| TI DM646x IBIS MODEL with DDR2
[IBIS Ver]   3.2
[File Name]   sprm277e.ibs
[File Rev]   0.2
[Date]   April 30, 2009
[Source]   TI
[Disclaimer]   Please be aware that in the absence of a written agreement
|   Texas Instruments(TI) assumes no liability for:
|   (1) The accuracy of the IBIS models provided to your company
|   (2) The proper functioning of these Models in your design
|   or for any resulting applications
|   (3) Infringement of patents, copyrights or intellectual
|   property rights resulting from your use of these
|   models.
|   TI provides IBIS Models as a service to our customers and
|   therefore reserves the right to limit distribution of the
|   Models.
[Copyright]   Property of Texas Instruments Incorporated.
|   Unauthorized reproduction and/or distribution is strictly.
|   prohibited.
|   This product is protected under copyright law and trade
|   secret law as an unpublished work.
|   Created 2007,(C) Copyright 1999-2007,
|   Texas Instruments Incorporated., All Rights Reserved.
|   These commodities are under the U.S. Government
|   distribution license control. As such,they are not to be
|   re-exported without the prior approval of the U.S.
|   Department of Commerce.
[Notes]
| Component   DM646x
[Component]   DM646x
[Manufacturer]   Texas Instruments
[Package]
| variable   typ   min   max
R_pkg   2.45454E-01   5.83181E-02   4.83686E-01
L_pkg   2.60207E-09   1.54140E-09   4.10250E-09
C_pkg   1.55780E-12   1.08555E-12   2.17328E-12
[Pin] signal_name   model_name   R_pin   L_pin   C_pin
A11   PCI_INTBN   BPCI33TPUFZP18   2.7877E-01 2.7673E-09 1.6313E-12
C11   PCI_INTAN   BPCI33TPUFZP18   1.8694E-01 2.2210E-09 1.3859E-12
D11   PCI_INTCN   BPCI33TPUFZP18   1.3871E-01 1.9025E-09 1.2538E-12
B11   GP05_INT05   BPCI33TPDFZP18   2.3300E-01 2.5519E-09 1.4959E-12
A12   GP07_INT07   BPCI33TPDFZP18   2.7619E-01 2.8667E-09 1.6467E-12
A10   PCI_CLK   BPCI33TPUFZP18   2.6854E-01 2.8128E-09 1.5917E-12
C10   PCI_RSTN   BPCI33TPDFZP18   1.5935E-01 2.1439E-09 1.3432E-12
B12   TCLK   IQ33STCKP18PUSR50   2.4188E-01 2.5826E-09 1.5351E-12
B10   PCI_REQ2N   BPCI33TPDFZP18   2.2910E-01 2.4910E-09 1.4928E-12
E11   GP06_INT06   BPCI33TPDFZP18   8.4748E-02 1.6414E-09 1.1002E-12
D12   TMS   IT33SHYPUFZP18   1.4649E-01 1.9445E-09 1.2763E-12
D10   PCI_GNTN   BPCI33TPUFZP18   1.5951E-01 2.0675E-09 1.3045E-12
E10   PCI_GNT2N   BPCI33TPUFZP18   9.3986E-02 1.6149E-09 1.1264E-12
E12   TRSTN   IT33SHYPDFZP18   1.1940E-01 1.7969E-09 1.2210E-12
C12   RTCK   OT3350CSFZP18   2.0113E-01 2.2992E-09 1.4287E-12
|C15  VSS_DEV   GND   5.5062E-02 1.6374E-09 1.9419E-12
B15   X1DEV_CKINDEV   NC   2.3651E-01 2.4675E-09 1.5117E-12
A15   X2DEV   NC   2.9679E-01 2.8758E-09 1.6904E-12
|D15  VDDS   POWER   7.5928E-02 1.7083E-09 1.8787E-12
|A16  VSSA2   GND   7.2873E-02 1.8878E-09 2.4529E-12
|C14  VSSA   GND   6.6017E-02 1.7036E-09 2.0833E-12
|C16  VSSS2   GND   6.3900E-02 1.5792E-09 1.9390E-12
|B14  VDDA18V   POWER   6.7389E-02 1.6921E-09 2.1872E-12
|D16  VDDS2   POWER   7.2580E-02 1.6472E-09 1.7765E-12
|B16  VDDA18V2   POWER   7.9345E-02 1.7827E-09 2.2027E-12
|C17  VSS_AUX   GND   8.3082E-02 1.7375E-09 1.9680E-12
B17   X1AUX_CKINAUX   NC   2.5695E-01 2.6223E-09 1.5724E-12
A17   X2AUX   NC   2.8397E-01 2.8078E-09 1.6441E-12
|E16  VDD5   POWER   9.4062E-02 1.6917E-09 1.5592E-12
D17   PORN   IT33SHYPUFZP18   1.7201E-01 2.1219E-09 1.3281E-12
C18   USB_VSSREF   NC   5.8318E-02 1.6295E-09 1.9812E-12
B18   USB_DRVVBUS   OPERATIONAL_MODE   2.5336E-01 2.7069E-09 1.6138E-12
|P23  VREF_DDR   POWER   4.9018E-02 1.3868E-09 7.8262E-12
N23   DDR_A14   BSHTLDVGPBFZIDID   2.8514E-01 2.8886E-09 1.6855E-12
N22   DDR_A09   BSHTLDVGPBFZIDID   2.2962E-01 2.4944E-09 1.5400E-12
N21   DDR_A05   BSHTLDVGPBFZIDID   1.9430E-01 2.3197E-09 1.4271E-12
R23   DDR_A01   BSHTLDVGPBFZIDID   3.7618E-01 3.6698E-09 1.8926E-12
Y21   DDR_D29   BSHTLDVGPBFZIDID   3.0072E-01 2.8974E-09 1.6783E-12
H22   DDR_D15   BSHTLDVGPBFZIDID   4.3087E-01 3.6600E-09 2.0046E-12
U20   DDR_DQS3   BSHTLDVGPBFZIDID   2.8732E-01 2.8089E-09 1.5764E-12
G22   DDR_D13   BSHTLDVGPBFZIDID   4.4213E-01 3.7401E-09 1.9738E-12
T23   DDR_A10   BSHTLDVGPBFZIDID   3.4959E-01 3.4591E-09 1.8147E-12
A2   THERMAL_P   NC   3.3115E-01 3.1439E-09 1.9476E-12
A1   THERMAL_N   NC   3.7687E-01 3.5180E-09 1.9528E-12
B3   PCI_DEVSELN   BPCI33TPUFZP18   3.0811E-01 2.9904E-09 1.7689E-12
A3   PCI_IRDYN   BPCI33TPUFZP18   3.6344E-01 3.2863E-09 1.8773E-12
C3   PCI_PERRN   BPCI33TPUFZP18   2.6286E-01 2.6646E-09 1.6213E-12
B2   PCI_SERRN   BPCI33TPUFZP18   2.8503E-01 2.8397E-09 1.7099E-12
D5   PCI_STOPN   BPCI33TPUFZP18   1.7666E-01 2.1759E-09 1.3763E-12
C1   PCI_AD14   BPCI33TPDFZP18   3.3204E-01 3.1677E-09 1.7799E-12
C4   PCI_CBE2N   BPCI33TPUFZP18   2.8951E-01 2.9542E-09 1.6700E-12
B4   PCI_AD17   BPCI33TPDFZP18   3.0308E-01 2.9750E-09 1.7299E-12
D4   PCI_PAR   BPCI33TPUFZP18   1.9363E-01 2.2404E-09 1.4282E-12
C2   PCI_CBE1N   BPCI33TPUFZP18   2.6565E-01 2.7844E-09 1.6478E-12
D2   PCI_AD10   BPCI33TPDFZP18   2.7296E-01 2.8166E-09 1.6458E-12
E5   PCI_AD15   BPCI33TPDFZP18   1.3925E-01 1.9027E-09 1.2655E-12
D3   PCI_AD12   BPCI33TPDFZP18   2.4623E-01 2.6009E-09 1.5479E-12
D6   PCI_FRAMEN   BPCI33TPUFZP18   1.8217E-01 2.2248E-09 1.3886E-12
C5   PCI_AD21   BPCI33TPDFZP18   2.8181E-01 2.8221E-09 1.6211E-12
C6   PCI_AD16   BPCI33TPDFZP18   2.1425E-01 2.4965E-09 1.4441E-12
E4   PCI_AD13   BPCI33TPDFZP18   1.6213E-01 2.0692E-09 1.3389E-12
E6   PCI_TRDYN   BPCI33TPUFZP18   1.0725E-01 1.7677E-09 1.1929E-12
A4   PCI_AD19   BPCI33TPDFZP18   3.8327E-01 3.4263E-09 1.9108E-12
E7   PCI_AD18   BPCI33TPDFZP18   1.2702E-01 1.7420E-09 1.2068E-12
D7   PCI_AD20   BPCI33TPDFZP18   1.5322E-01 2.0190E-09 1.2765E-12
F5   PCI_AD9   BPCI33TPDFZP18   1.4050E-01 1.9648E-09 1.2543E-12
C7   PCI_AD22   BPCI33TPDFZP18   1.8238E-01 2.1596E-09 1.4090E-12
B5   PCI_AD23   BPCI33TPDFZP18   2.9356E-01 2.8622E-09 1.7076E-12
B6   PCI_AD25   BPCI33TPDFZP18   2.9546E-01 2.8485E-09 1.7200E-12
A5   PCI_CBE3N   BPCI33TPUFZP18   3.6680E-01 3.3978E-09 1.9010E-12
E8   PCI_IDSEL   BPCI33TPUFZP18   1.2603E-01 1.8511E-09 1.2174E-12
D8   PCI_AD24   BPCI33TPDFZP18   1.4545E-01 1.9034E-09 1.2897E-12
C8   PCI_AD26   BPCI33TPDFZP18   1.9932E-01 2.2035E-09 1.4169E-12
B8   PCI_AD29   BPCI33TPDFZP18   2.2504E-01 2.4923E-09 1.5032E-12
A6   PCI_AD27   BPCI33TPDFZP18   3.4528E-01 3.2406E-09 1.8202E-12
E9   PCI_GNT1N   BPCI33TPDFZP18   1.0641E-01 1.7227E-09 1.1832E-12
D9   PCI_AD28   BPCI33TPDFZP18   1.7577E-01 2.1341E-09 1.3584E-12
C9   PCI_AD30   BPCI33TPDFZP18   1.9116E-01 2.2644E-09 1.3919E-12
A8   PCI_AD31   BPCI33TPDFZP18   2.9816E-01 2.8914E-09 1.6888E-12
B9   PCI_REQN   BPCI33TPUFZP18   2.2823E-01 2.4067E-09 1.5054E-12
A9   PCI_REQ1N   BPCI33TPDFZP18   2.4922E-01 2.7180E-09 1.5936E-12
A13   EMU0   BT3350CSHYPUFZP18   2.8486E-01 2.8884E-09 1.6409E-12
B13   EMU1   BT3350CSHYPUFZP18   2.5408E-01 2.7080E-09 1.5863E-12
C13   CLKOUT0   OT3350BSFZP18   2.1075E-01 2.5326E-09 1.4228E-12
D13   TDO   OT3350CSFZP18   1.9701E-01 2.3477E-09 1.4279E-12
E13   TDI   IT33SHYPUFZP18   1.2685E-01 1.9618E-09 1.2659E-12
D14   AMUX   NC   6.0907E-02 1.5939E-09 1.7516E-12
|E14  VSSS1   GND   5.5579E-02 1.5715E-09 1.4300E-12
|E15  VDD6   POWER   6.3533E-02 1.5903E-09 1.5396E-12
A19   USB_DP   DPDM   2.9913E-01 2.8266E-09 1.7243E-12
|E17  VDDA_12LDO   POWER   4.8724E-02 1.4146E-09 1.4594E-12
|G16  VPP   POWER   1.4716E-02 9.8859E-10 2.0313E-12
D18   USB_R1   NC   1.7146E-01 2.1995E-09 1.3651E-12
C20   DDR_D02   BSHTLDVGPBFZIDID   3.7216E-01 3.2805E-09 1.7796E-12
A20   USB_DN   DPDM   2.9706E-01 2.8346E-09 1.7381E-12
D20   DDR_D01   BSHTLDVGPBFZIDID   3.3792E-01 3.1510E-09 1.7608E-12
|E18  VDD_18UPHY   POWER   5.6087E-02 1.5095E-09 1.5146E-12
|F18  VDDA_33UPHY   POWER   3.8147E-02 1.3788E-09 1.3634E-12
F20   DDR_DQM0   BSHTLDVGPBFZIDID   3.4058E-01 3.0257E-09 1.7935E-12
A22   IFORCE   NC   3.8507E-01 3.4309E-09 1.9972E-12
B21   DDR_D03   BSHTLDVGPBFZIDID   3.8767E-01 3.4318E-09 1.9469E-12
G20   DDR_D04   BSHTLDVGPBFZIDID   3.4303E-01 3.0700E-09 1.7241E-12
E20   DDR_DQSN0   BSHTLDVGPBFZIDID   3.5451E-01 3.1555E-09 1.7460E-12
A23   VSENSE   NC   4.3154E-01 3.8929E-09 2.0758E-12
C21   DDR_D00   BSHTLDVGPBFZIDID   3.8272E-01 3.2914E-09 1.8910E-12
B22   DDR_D09   BSHTLDVGPBFZIDID   4.8369E-01 4.1025E-09 2.1733E-12
C23   DDR_D08   BSHTLDVGPBFZIDID   4.3765E-01 3.7508E-09 2.0793E-12
C22   DDR_D10   BSHTLDVGPBFZIDID   4.3926E-01 3.6854E-09 2.0784E-12
J19   DDR_DQGATE0   BSHTLDVGPBFZIDID   1.3943E-01 1.8775E-09 1.2336E-12
D21   DDR_DQS0   BSHTLDVGPBFZIDID   3.5612E-01 3.2791E-09 1.8411E-12
F21   DDR_D05   BSHTLDVGPBFZIDID   3.5077E-01 3.1080E-09 1.8262E-12
G21   DDR_D06   BSHTLDVGPBFZIDID   3.4698E-01 3.1246E-09 1.7646E-12
D22   DDR_DQS1   BSHTLDVGPBFZIDID   4.4339E-01 3.7215E-09 2.1383E-12
H20   DDR_D07   BSHTLDVGPBFZIDID   3.4601E-01 3.0269E-09 1.7012E-12
J21   DDR_DQGATE1   BSHTLDVGPBFZIDID   1.6504E-01 2.1300E-09 1.3912E-12
H21   DDR_A13   BSHTLDVGPBFZIDID   2.6986E-01 2.7281E-09 1.6286E-12
F22   DDR_DQM1   BSHTLDVGPBFZIDID   4.2218E-01 3.5920E-09 2.0151E-12
J20   DDR_CSN   BSHTLDVGPBFZIDID   2.0809E-01 2.4992E-09 1.5659E-12
K20   DDR_ODT0   BSHTLDVGPBFZIDID   1.3671E-01 1.9192E-09 1.2745E-12
K19   DDR_RASN   BSHTLDVGPBFZIDID   1.3844E-01 2.0285E-09 1.3514E-12
J22   DDR_A04   BSHTLDVGPBFZIDID   2.5719E-01 2.6382E-09 1.6209E-12
D23   DDR_DQSN1   BSHTLDVGPBFZIDID   4.4173E-01 3.6954E-09 2.1371E-12
E23   DDR_D11   BSHTLDVGPBFZIDID   4.3505E-01 3.7028E-09 1.9933E-12
F23   DDR_D12   BSHTLDVGPBFZIDID   4.4355E-01 3.6991E-09 2.0659E-12
G23   DDR_D14   BSHTLDVGPBFZIDID   4.2279E-01 3.7370E-09 2.0122E-12
H23   DDR_A00   BSHTLDVGPBFZIDID   3.1449E-01 3.0248E-09 1.7505E-12
J23   DDR_A08   BSHTLDVGPBFZIDID   3.4902E-01 3.3817E-09 1.8271E-12
L20   DDR_WEN   BSHTLDVGPBFZIDID   1.7445E-01 2.1296E-09 1.3326E-12
L21   DDR_CASN   BSHTLDVGPBFZIDID   1.9727E-01 2.2693E-09 1.4121E-12
L19   DDR_REFP   NC   1.3252E-01 2.1619E-09 1.2826E-12
K23   DDR_A11   BSHTLDVGPBFZIDID   2.7410E-01 2.7849E-09 1.6432E-12
M22   DDR_A06   BSHTLDVGPBFZIDID   2.3631E-01 2.6236E-09 1.5578E-12
L22   DDR_A02   BSHTLDVGPBFZIDID   2.4786E-01 2.9281E-09 1.5341E-12
M21   DDR_BA1   BSHTLDVGPBFZIDID   1.7634E-01 2.2453E-09 1.3659E-12
M20   DDR_CKE   BSHTLDVGPBFZIDID   1.6773E-01 2.1873E-09 1.3066E-12
L23   DDR_CLKN   BSHTLDVGPBFZIDID   2.9719E-01 3.0043E-09 1.6909E-12
M23   DDR_CLK   BSHTLDVGPBFZIDID   2.9064E-01 2.8534E-09 1.7072E-12
M19   DDR_REFN   NC   9.8133E-02 1.6910E-09 1.1266E-12
R22   DDR_A03   BSHTLDVGPBFZIDID   2.7119E-01 2.8434E-09 1.6357E-12
T22   DDR_D17   BSHTLDVGPBFZIDID   3.9328E-01 3.4903E-09 1.9637E-12
N19   DDR_BA0   BSHTLDVGPBFZIDID   7.9436E-02 1.5414E-09 1.0856E-12
N20   DDR_A07   BSHTLDVGPBFZIDID   1.3620E-01 2.0966E-09 1.2215E-12
P20   DDR_A12   BSHTLDVGPBFZIDID   1.4662E-01 1.9794E-09 1.2429E-12
R21   DDR_DQGATE3   BSHTLDVGPBFZIDID   1.9255E-01 2.2141E-09 1.3949E-12
U23   DDR_D18   BSHTLDVGPBFZIDID   4.0960E-01 3.6369E-09 1.9140E-12
U22   DDR_D16   BSHTLDVGPBFZIDID   4.2102E-01 3.8021E-09 1.9612E-12
P19   DDR_BA2   BSHTLDVGPBFZIDID   1.4495E-01 2.0123E-09 1.2598E-12
R19   DDR_DQGATE2   BSHTLDVGPBFZIDID   1.4044E-01 1.8898E-09 1.1869E-12
R20   DDR_D25   BSHTLDVGPBFZIDID   2.8920E-01 2.7835E-09 1.6410E-12
Y23   DDR_DQM2   BSHTLDVGPBFZIDID   4.4716E-01 4.0407E-09 2.1157E-12
T21   DDR_D26   BSHTLDVGPBFZIDID   2.8616E-01 2.7532E-09 1.6110E-12
AA23  DDR_D20   BSHTLDVGPBFZIDID   4.4661E-01 3.9010E-09 2.1348E-12
W23   DDR_DQSN2   BSHTLDVGPBFZIDID   4.1680E-01 3.6580E-09 2.0554E-12
Y22   DDR_D22   BSHTLDVGPBFZIDID   4.1015E-01 3.5365E-09 2.0298E-12
AA22  DDR_D21   BSHTLDVGPBFZIDID   4.5800E-01 4.0009E-09 2.1196E-12
V23   DDR_D19   BSHTLDVGPBFZIDID   4.0434E-01 3.6008E-09 1.9715E-12
V22   DDR_DQS2   BSHTLDVGPBFZIDID   4.1978E-01 3.6565E-09 1.9620E-12
U21   DDR_D27   BSHTLDVGPBFZIDID   2.9025E-01 2.7701E-09 1.6060E-12
V21   DDR_DQSN3   BSHTLDVGPBFZIDID   2.8454E-01 2.6807E-09 1.6218E-12
AB22  DDR_D23   BSHTLDVGPBFZIDID   4.5536E-01 4.0091E-09 2.1416E-12
AA21  DDR_D28   BSHTLDVGPBFZIDID   3.2699E-01 3.0902E-09 1.6728E-12
AC21  UART2_CTSN   BT3350BSHYPUFZP18   3.3320E-01 3.1564E-09 1.7751E-12
T20   DDR_D24   BSHTLDVGPBFZIDID   2.8107E-01 2.8430E-09 1.6321E-12
V20   DDR_DQM3   BSHTLDVGPBFZIDID   2.9327E-01 2.7837E-09 1.6108E-12
W20   DDR_D30   BSHTLDVGPBFZIDID   2.8787E-01 2.8040E-09 1.6332E-12
Y20   DDR_D31   BSHTLDVGPBFZIDID   2.9876E-01 2.8963E-09 1.6159E-12
AB20  UART2_RXD   OPERATIONAL_MODE   2.6882E-01 2.8323E-09 1.6277E-12
Y18   UART1_RXD   OPERATIONAL_MODE   1.5530E-01 1.9932E-09 1.3127E-12
AA19  UART2_TXD   OPERATIONAL_MODE   2.2431E-01 2.4176E-09 1.4946E-12
W18   PWM1   OT3350BSFZP18   8.4804E-02 1.6219E-09 1.1306E-12
W17   PWM0   OT3350BSFZP18   9.0402E-02 1.5786E-09 1.1118E-12
Y17   UART1_CTSN   BT3350BSHYPUFZP18   1.4102E-01 1.9809E-09 1.2447E-12
Y16   VPIF_DIN11   BT3350DSHYPDFZSCP18  1.4363E-01 1.9195E-09 1.3669E-12
AC20  UART2_RTSN   BT3350BSHYPUFZP18   3.4151E-01 3.2147E-09 1.8048E-12
Y15   VPIF_DIN3   BT3350DSHYPDFZSCP18  1.3560E-01 1.8601E-09 1.2381E-12
AC19  PTSI_CLK   BT3350DSHYPDFZSCP18  3.2733E-01 3.0457E-09 1.7567E-12
AB19  UART1_TXD   OPERATIONAL_MODE   2.7053E-01 2.7661E-09 1.6006E-12
AC18  VPIF_DIN15_VSYNC   BT3350DSHYPDFZSCP18  2.7932E-01 2.8561E-09 1.6429E-12
AA18  UART1_RTSN   BT3350BSHYPUFZP18   1.8570E-01 2.2909E-09 1.3928E-12
AB18  VPIF_CLKIN1   BT3350DSHYPDFZSCP18  2.4542E-01 2.6350E-09 1.5337E-12
AA17  VPIF_DIN14_HSYNC   BT3350DSHYPDFZSCP18  1.9262E-01 2.3298E-09 1.3637E-12
AB17  VPIF_DIN13_FIELD   BT3350DSHYPDFZSCP18  2.5132E-01 2.7150E-09 1.5596E-12
AC17  VPIF_DIN12   BT3350DSHYPDFZSCP18  2.6084E-01 2.7842E-09 1.6075E-12
AA16  VPIF_DIN10   BT3350DSHYPDFZSCP18  1.9516E-01 2.4361E-09 1.3961E-12
AC16  VPIF_DIN8   BT3350DSHYPDFZSCP18  2.6928E-01 2.7639E-09 1.6996E-12
AB16  VPIF_DIN9   BT3350DSHYPDFZSCP18  2.1019E-01 2.4044E-09 1.4676E-12
AA15  VPIF_DIN2   BT3350DSHYPDFZSCP18  1.6289E-01 2.1339E-09 1.4187E-12
AB15  VPIF_DIN1   BT3350DSHYPDFZSCP18  2.2152E-01 2.4260E-09 1.4881E-12
AC15  VPIF_DIN0   BT3350DSHYPDFZSCP18  2.7519E-01 2.7685E-09 1.7276E-12
Y14   VPIF_DIN7   BT3350DSHYPDFZSCP18  1.2325E-01 1.8854E-09 1.2171E-12
AA14  VPIF_DIN6   BT3350DSHYPDFZSCP18  1.9104E-01 2.2307E-09 1.3836E-12
AB14  VPIF_DIN5   BT3350DSHYPDFZSCP18  2.2322E-01 2.4590E-09 1.4752E-12
AC14  VPIF_DIN4   BT3350DSHYPDFZSCP18  2.4866E-01 2.6792E-09 1.5862E-12
AC13  VPIF_CLKIN0   BT3350DSHYPDFZSCP18  2.5976E-01 2.5128E-09 1.6572E-12
AB13  UART0_RXD   IT33SHYPDFZP18   2.1891E-01 2.4350E-09 1.5402E-12
AA13  UART0_RTSN   BT3350BSHYPUFZP18   1.7651E-01 2.1599E-09 1.3503E-12
Y13   UART0_TXD   OPERATIONAL_MODE   1.1551E-01 1.7462E-09 1.1995E-12
AC12  UART0_CTSN   BT3350BSHYPUFZP18   2.7766E-01 2.6877E-09 1.6259E-12
AB11  UART0_DSRN   BT3350BSHYPUFZP18   2.4043E-01 2.4347E-09 1.5251E-12
AA11  UART0_DCDN   BT3350BSHYPUFZP18   1.7124E-01 2.0643E-09 1.3628E-12
AC11  STSI_CLK   BT3350DSHYPDFZSCP18  2.5839E-01 2.6519E-09 1.6141E-12
Y12   UART0_DTRN   BT3350BSHYPUFZP18   1.4024E-01 1.8911E-09 1.2584E-12
AC10  VPIF_CLKO3   OT3350CSFZP18   2.7995E-01 2.7900E-09 1.6256E-12
AB10  VPIF_DOUT11   BT3350DSHYPDFZSCP18  2.3455E-01 2.4754E-09 1.5331E-12
Y11   UART0_RIN   OPERATIONAL_MODE   1.4936E-01 1.9491E-09 1.2751E-12
AA10  VPIF_DOUT10   BT3350DSHYPDFZSCP18  2.0346E-01 2.3261E-09 1.5218E-12
Y10   VPIF_CLKIN2   BT3350DSHYPDFZSCP18  1.2823E-01 1.8376E-09 1.3732E-12
AC9   VPIF_CLKIN3   BT3350DSHYPDFZSCP18  2.9240E-01 2.8708E-09 1.6918E-12
AB9   VPIF_DOUT8   BT3350DSHYPDFZSCP18  2.4640E-01 2.6076E-09 1.6771E-12
AC8   VPIF_DOUT9   BT3350DSHYPDFZSCP18  2.9478E-01 2.9570E-09 1.7786E-12
AB8   VPIF_DOUT15   BT3350DSHYPDFZSCP18  2.5729E-01 2.6739E-09 1.6805E-12
AA9   VPIF_CLKO2   OT3350CSFZP18   2.2390E-01 2.4214E-09 1.6053E-12
Y9   VPIF_DOUT13   BT3350DSHYPDFZSCP18  1.4080E-01 1.9714E-09 1.4233E-12
AC7   VPIF_DOUT14   BT3350DSHYPDFZSCP18  3.1034E-01 3.0264E-09 1.8146E-12
AB7   VPIF_DOUT7   BT3350DSHYPDFZSCP18  2.7625E-01 2.8729E-09 1.6145E-12
AA8   VPIF_DOUT12   BT3350DSHYPDFZSCP18  2.0748E-01 2.2980E-09 1.4394E-12
Y8   VPIF_DOUT2_BTMODE2 BT3350DSHYPDFZSCP18  1.5979E-01 2.0654E-09 1.2868E-12
W8   TOUT0   OPERATIONAL_MODE   1.2111E-01 1.8172E-09 1.1672E-12
AC6   VPIF_DOUT5_PCIEN   BT3350DSHYPDFZSCP18  3.2373E-01 3.1423E-09 1.7568E-12
AB6   VPIF_DOUT3_BTMODE3 BT3350DSHYPDFZSCP18  2.6945E-01 2.7674E-09 1.6270E-12
AA7   VPIF_DOUT4_CS2BW   BT3350DSHYPDFZSCP18  2.3870E-01 2.5626E-09 1.5246E-12
Y7   TIN0   OPERATIONAL_MODE   1.7576E-01 2.1685E-09 1.3360E-12
AC5   VPIF_DOUT6_DSPBOOT BT3350DSHYPDFZSCP18  3.3354E-01 3.1744E-09 1.8243E-12
AA6   TIN1   OPERATIONAL_MODE   2.1716E-01 2.4245E-09 1.4749E-12
AC4   VPIF_DOUT1_BTMODE1 BT3350DSHYPDFZSCP18  3.5677E-01 3.3407E-09 1.8479E-12
AB5   VPIF_DOUT0_BTMODE0 BT3350DSHYPDFZSCP18  2.8554E-01 2.8645E-09 1.6703E-12
AB4   TOUT3   OPERATIONAL_MODE   2.9729E-01 3.0600E-09 1.6692E-12
Y6   TIN2   OPERATIONAL_MODE   1.7426E-01 2.2147E-09 1.3603E-12
W7   TOUT1   OPERATIONAL_MODE   1.5461E-01 2.0530E-09 1.2905E-12
AA5   TOUT2   OPERATIONAL_MODE   2.4354E-01 2.6342E-09 1.5345E-12
AA4   GP02_INT02   OPERATIONAL_MODE   2.5812E-01 2.7070E-09 1.5900E-12
AC3   GP04_INT04   OPERATIONAL_MODE   3.7246E-01 3.4943E-09 1.8744E-12
AB3   GP03_INT03   OPERATIONAL_MODE   3.1393E-01 2.9942E-09 1.7522E-12
W6   RESETN   IT33SHYPUFZP18   1.7245E-01 2.1287E-09 1.2881E-12
Y5   TOUT4   OPERATIONAL_MODE   1.9436E-01 2.3107E-09 1.4284E-12
Y4   MCA0_AFSX   OPERATIONAL_MODE   2.1135E-01 2.3148E-09 1.4788E-12
W5   GP00_INT00   OPERATIONAL_MODE   1.5172E-01 1.9685E-09 1.3059E-12
W4   MCA0_AXR2   OPERATIONAL_MODE   1.8296E-01 2.1469E-09 1.3810E-12
V5   GP01_INT01   OPERATIONAL_MODE   1.6559E-01 2.2628E-09 1.3157E-12
AB2   MCA0_AHCLKR   OPERATIONAL_MODE   3.7868E-01 3.4051E-09 1.9200E-12
AA2   MCA0_ACLKR   OPERATIONAL_MODE   3.4985E-01 3.3208E-09 1.8166E-12
AA3   MCA0_AMUTEIN   IT33SHYPDFZP18   2.6275E-01 2.6658E-09 1.5867E-12
V4   MCA0_AXR1   OPERATIONAL_MODE   1.5577E-01 1.9983E-09 1.3178E-12
U5   IIC_SCL   BI2CSFZP18   1.2580E-01 1.7894E-09 1.2346E-12
U4   IIC_SDA   BI2CSFZP18   1.6630E-01 2.1408E-09 1.3229E-12
AA1   MCA0_ACLKX   OPERATIONAL_MODE   3.4948E-01 3.1808E-09 1.8434E-12
Y2   MCA0_AMUTE   OPERATIONAL_MODE   2.8818E-01 2.8337E-09 1.6831E-12
Y1   MCA0_AHCLKX   OPERATIONAL_MODE   2.8499E-01 2.8404E-09 1.6822E-12
Y3   MCA0_AFSR   OPERATIONAL_MODE   2.3291E-01 2.5316E-09 1.5548E-12
W3   MCA0_AXR3   OPERATIONAL_MODE   1.9293E-01 2.2021E-09 1.4279E-12
W2   MCA1_AHCLKX   OPERATIONAL_MODE   2.6844E-01 2.7111E-09 1.6166E-12
W1   MCA1_ACLKX   OPERATIONAL_MODE   2.9748E-01 2.8653E-09 1.6952E-12
V2   MCA1_AXR0   OPERATIONAL_MODE   2.2999E-01 2.5334E-09 1.5258E-12
V3   MCA0_AXR0   OPERATIONAL_MODE   1.8338E-01 2.2344E-09 1.3914E-12
U3   SPI_SCS1   OPERATIONAL_MODE   1.9911E-01 2.3738E-09 1.4037E-12
V1   SPI_SCLK   BT3350DSHYPDFZSCP18  2.7473E-01 2.8949E-09 1.6383E-12
U2   VLNQ_SCRUN   BT3350DSHYPUFZSCP18  2.4837E-01 2.6343E-09 1.5512E-12
U1   VLNQ_CLOCK   BT3350DSHYPUFZSCP18  2.7156E-01 2.8034E-09 1.6497E-12
T5   SPI_EN   OPERATIONAL_MODE   9.6016E-02 1.6996E-09 1.1385E-12
T4   SPI_SCS0   OPERATIONAL_MODE   1.2694E-01 1.8952E-09 1.2360E-12
T2   VLNQ_TXD2   OT3350DSFZSCP18   2.1964E-01 2.5063E-09 1.4934E-12
R5   SPI_MISO   OPERATIONAL_MODE   8.7907E-02 1.5584E-09 1.1049E-12
R4   VLNQ_TXD0   OT3350DSFZSCP18   1.6528E-01 2.0956E-09 1.3209E-12
T3   VLNQ_TXD3   OT3350DSFZSCP18   2.0131E-01 2.2969E-09 1.4209E-12
R3   VLNQ_RXD3   IT33SHYPDFZP18   1.7122E-01 2.1551E-09 1.3668E-12
P5   SPI_MOSI   OPERATIONAL_MODE   1.0539E-01 1.8190E-09 1.1520E-12
P4   VLNQ_RXD0   IT33SHYPDFZP18   1.2412E-01 1.8656E-09 1.2238E-12
N4   MII_MTXD6   OT3325ESFZSCP18   1.2865E-01 1.8605E-09 1.2315E-12
M4   MII_MTXD2   OT3325ESFZSCP18   1.3680E-01 1.9323E-09 1.2413E-12
T1   VLNQ_TXD1   OT3350DSFZSCP18   2.7833E-01 2.8178E-09 1.6319E-12
R2   VLNQ_RXD2   IT33SHYPDFZP18   2.3872E-01 2.4894E-09 1.5361E-12
R1   MII_MTCLK   IT33SHYPDFZP18   2.7549E-01 2.8126E-09 1.6302E-12
P3   VLNQ_RXD1   IT33SHYPDFZP18   1.9149E-01 2.2530E-09 1.4022E-12
P2   MII_GMTCLK   OT3325ESFZSCP18   2.2041E-01 2.4009E-09 1.4812E-12
P1   MII_MTXD7   OT3325ESFZSCP18   2.4813E-01 2.6646E-09 1.5719E-12
N3   MII_MTXD5   OT3325ESFZSCP18   1.8028E-01 2.2355E-09 1.3788E-12
N2   MII_MTXD4   OT3325ESFZSCP18   2.0075E-01 2.3299E-09 1.4530E-12
N1   MII_MTXD3   OT3325ESFZSCP18   2.5900E-01 2.7740E-09 1.5893E-12
L3   MII_MCRS   IT33SHYPDFZP18   1.7399E-01 2.1256E-09 1.3621E-12
M1   MII_MTXD1   OT3325ESFZSCP18   2.5068E-01 2.6600E-09 1.5519E-12
L2   MII_MTXEN   OT3325ESFZSCP18   2.1371E-01 2.3315E-09 1.4669E-12
L4   MII_MCOL   IT33SHYPDFZP18   1.1398E-01 1.8135E-09 1.2070E-12
L1   MII_MTXD0   OT3325ESFZSCP18   2.4024E-01 2.5084E-09 1.5524E-12
K1   MII_MRCLK   IT33SHYPUFZP18   2.7303E-01 2.7547E-09 1.6145E-12
K2   MII_MRXD7   IT33SHYPUFZP18   2.0415E-01 2.3013E-09 1.4440E-12
K3   MII_MRXD6   IT33SHYPUFZP18   1.7847E-01 2.1246E-09 1.3445E-12
K4   MII_MRXD5   IT33SHYPUFZP18   1.3799E-01 1.8787E-09 1.2336E-12
J3   MII_MRXD2   IT33SHYPUFZP18   1.9714E-01 2.2803E-09 1.4227E-12
J1   MII_MRXD4   IT33SHYPUFZP18   2.5650E-01 2.6839E-09 1.5977E-12
J2   MII_MRXD3   IT33SHYPUFZP18   2.2986E-01 2.4807E-09 1.5096E-12
J4   MII_MRXDV   IT33SHYPUFZP18   1.2298E-01 1.8239E-09 1.2001E-12
H1   MII_RFTCLK   IT33SHYPDFZP18   2.6959E-01 2.7493E-09 1.6518E-12
H2   MII_MRXD1   IT33SHYPUFZP18   2.3833E-01 2.4865E-09 1.5254E-12
H3   MII_MRXER   IT33SHYPUFZP18   1.9422E-01 2.2555E-09 1.4000E-12
H4   MDIO_MDIO   BC3350BSHYPUFZP18   1.4184E-01 1.9320E-09 1.2849E-12
G1   MDIO_MDCLK   BC3350BSHYPUFZP18   2.9520E-01 2.9301E-09 1.6865E-12
G2   MII_MRXD0   IT33SHYPUFZP18   2.6805E-01 2.7049E-09 1.5901E-12
G3   PCI_AD0   BPCI33TPDFZP18   2.1670E-01 2.6112E-09 1.4303E-12
F2   PCI_AD3   BPCI33TPDFZP18   2.6339E-01 2.6476E-09 1.5905E-12
F3   PCI_AD6   BPCI33TPDFZP18   2.0672E-01 2.4545E-09 1.4259E-12
G4   PCI_AD2   BPCI33TPDFZP18   1.6718E-01 2.2180E-09 1.3471E-12
F1   PCI_AD1   BPCI33TPDFZP18   3.1470E-01 3.0675E-09 1.7331E-12
G5   PCI_AD4   BPCI33TPDFZP18   1.3002E-01 1.8846E-09 1.2535E-12
E1   PCI_AD5   BPCI33TPDFZP18   3.0120E-01 3.0221E-09 1.7174E-12
E2   PCI_AD7   BPCI33TPDFZP18   2.7202E-01 2.8695E-09 1.6020E-12
E3   PCI_AD11   BPCI33TPDFZP18   2.1768E-01 2.5498E-09 1.4652E-12
F4   PCI_CBE0N   BPCI33TPUFZP18   1.6625E-01 2.2058E-09 1.3301E-12
D1   PCI_AD8   BPCI33TPDFZP18   3.1798E-01 3.1283E-09 1.7313E-12
[Diff Pin] inv_pin vdiff tdelay_typ tdelay_min tdelay_max
A19   A20   0   1nS   NA   NA
M23   L23   0   1nS   NA   NA
|In model selector :
|  IND TEMP means Industrial temperature ( -40 - 125 deg. C)
|  COM TEMP means Commercial temperature (   0 - 105 deg. C)
[Model Selector] BC3350BSHYPUFZP18
HYPUFZP18_M2_IND_3P3  Cell operated at 3.3(nom) IND TEMP with pullup on
HYPUFZP18_M1_IND_3P3  Cell operated at 3.3(nom) IND TEMP with pullup off
HYPUFZP18_M2_COM_3P3  Cell operated at 3.3(nom) COM TEMP with pullup on
HYPUFZP18_M1_COM_3P3  Cell operated at 3.3(nom) COM TEMP with pullup off
[Model Selector] BI2CSFZP18
BI2CSFZP18_COM_3P3  Cell operated at 3.3(nom) COM TEMP MODE
BI2CSFZP18_IND_3P3  Cell operated at 3.3(nom) IND TEMP MODE
[Model Selector] BPCI33TPDFZP18
3TPDFZP18_M2_COM_3P3  Cell operated at 3.3(nom) COM TEMP with pulldown on
3TPDFZP18_M1_COM_3P3  Cell operated at 3.3(nom) COM TEMP with pulldown off
3TPDFZP18_M2_IND_3P3  Cell operated at 3.3(nom) IND TEMP with pulldown on
3TPDFZP18_M1_IND_3P3  Cell operated at 3.3(nom) IND TEMP with pulldown off
[Model Selector] BPCI33TPUFZP18
3TPUFZP18_M2_COM_3P3  Cell operated at 3.3(nom) COM TEMP with pullup on
3TPUFZP18_M1_COM_3P3  Cell operated at 3.3(nom) COM TEMP with pullup off
3TPUFZP18_M2_IND_3P3  Cell operated at 3.3(nom) IND TEMP with pullup on
3TPUFZP18_M1_IND_3P3  Cell operated at 3.3(nom) IND TEMP with pullup off
[Model Selector]   OPERATIONAL_MODE
HYPDFZP18_M2_IND_3P3  Cell operated at 3.3(nom) IND TEMP WITH PULLDOWN ON
HYPDFZP18_M1_IND_3P3  Cell operated at 3.3(nom) IND TEMP WITH PULLDOWN OFF
HYPDFZP18_M2_COM_3P3  Cell operated at 3.3(nom) COM TEMP WITH PULLDOWN ON
HYPDFZP18_M1_COM_3P3  Cell operated at 3.3(nom) COM TEMP WITH PULLDOWN OFF
[Model Selector]   BT3350BSHYPUFZP18
BT3350BSHYPUFZP18_Z   Pullup_Off
BT3350BSHYPUFZP18_PU   Pullup_On
[Model Selector] BT3350CSHYPUFZP18
BCHYPUFZP18M2IND3P3  Cell operated at 3.3(nom) IND TEMP with pullup on
BCHYPUFZP18M1IND3P3  Cell operated at 3.3(nom) IND TEMP pullup off
BCHYPUFZP18M2COM3P3  Cell operated at 3.3(nom) COM TEMP with pullup on
BCHYPUFZP18M1COM3P3  Cell operated at 3.3(nom) COM TEMP pullup off
[Model Selector] BT3350DSHYPDFZSCP18
PDFZSCP18_M1_IND_3P3  Cell operated at 3.3(nom) IND TEMP WITH PULLDOWN ON
PDFZSCP18_M5_IND_3P3  Cell operated at 3.3(nom) IND TEMP WITH PULLDOWN OFF
PDFZSCP18_M1_COM_3P3  Cell operated at 3.3(nom) COM TEMP WITH PULLDOWN ON
PDFZSCP18_M5_COM_3P3  Cell operated at 3.3(nom) COM TEMP WITH PULLDOWN OFF
[Model Selector] BT3350DSHYPUFZSCP18
PUFZSCP18_M1_IND_3P3  Cell operated at 3.3(nom) IND TEMP WITH PULLUP ON
PUFZSCP18_M5_IND_3P3  Cell operated at 3.3(nom) IND TEMP WITH PULLUP OFF
PUFZSCP18_M1_COM_3P3  Cell operated at 3.3(nom) COM TEMP WITH PULLUP ON
PUFZSCP18_M5_COM_3P3  Cell operated at 3.3(nom) COM TEMP WITH PULLUP OFF
[Model Selector] DPDM
FS FS mode
LS LS mode
HS HS mode|
[Model Selector] FSLS_IN
FS_IN FS mode
LS_IN LS mode
[Model Selector] IQ33STCKP18PUSR50
KP18PUSR50_MODE2_M1  Cell operated at 3.3V & IND temp with Pullup On
KP18PUSR50_MODE1_M1  Cell operated at 3.3V & IND temp with Pullup Off
KP18PUSR50_MODE2_M2  Cell operated at 3.3V & COM temp with Pullup On
KP18PUSR50_MODE1_M2  Cell operated at 3.3V & COM temp with Pullup Off
[Model Selector] IT33SHYPDFZP18
SHYPDFZP18_MODE2_M1  Cell operated at 3.3V & IND temp with Pulldown On
SHYPDFZP18_MODE1_M1  Cell operated at 3.3V & IND temp with Pulldown Off
SHYPDFZP18_MODE2_M2  Cell operated at 3.3V & COM temp with Pulldown On
SHYPDFZP18_MODE1_M2  Cell operated at 3.3V & COM temp with Pulldown Off
[Model Selector] IT33SHYPUFZP18
SHYPUFZP18_MODE2_M1  Cell operated at 3.3V & IND temp with Pullup On
SHYPUFZP18_MODE1_M1  Cell operated at 3.3V & IND temp with Pullup Off
SHYPUFZP18_MODE2_M2  Cell operated at 3.3V & COM temp with Pullup On
SHYPUFZP18_MODE1_M2  Cell operated at 3.3V & COM temp with Pullup Off
[Model Selector] OT3325ESFZSCP18
BUF_MODE3_3P3_IND  Cell operated at 3.3V & IND temp
BUF_MODE3_3P3_COM  Cell operated at 3.3V & COM temp
[Model Selector] OT3350BSFZP18
OT3350BSFZP18_M1  Cell operated at 3.3V & IND temp - Default Mode
OT3350BSFZP18_M2  Cell operated at 3.3V & COM temp - Default Mode
[Model Selector] OT3350CSFZP18
OT3350CSFZP18_M1  Cell operated at 3.3V & IND temp - Default Mode
OT3350CSFZP18_M2  Cell operated at 3.3V & COM temp - Default Mode
[Model Selector] OT3350DSFZSCP18
BUF8_MODE1_3P3_IND  Cell operated at 3.3V & IND temp - Default Mode
BUF8_MODE1_3P3_COM  Cell operated at 3.3V & COM temp - Default Mode
[Model Selector] BSHTLDVGPBFZIDID
NO_SR0_NO_TERM_1P8  Cell operated at 1.8(nom)
|Driver model in Fast Mode of operation, 1P8V +/-5% Operation
NO_TERM_1P8  Cell operated at 1.8(nom)
|Reciever in No Termination Mode, 1P8V +/-5% Operation
SR0_NO_TERM_1P8  Cell operated at 1.8(nom)
| Models and submodels in the file (60): HYPUFZP18_M2_IND_3P3 (I/O), HYPUFZP18_M1_IND_3P3 (I/O), HYPUFZP18_M2_COM_3P3 (I/O), HYPUFZP18_M1_COM_3P3 (I/O), BI2CSFZP18_COM_3P3 (I/O_open_drain), BI2CSFZP18_IND_3P3 (I/O_open_drain), 3TPDFZP18_M2_COM_3P3 (I/O), 3TPDFZP18_M1_COM_3P3 (I/O), 3TPDFZP18_M2_IND_3P3 (I/O), 3TPDFZP18_M1_IND_3P3 (I/O), 3TPUFZP18_M2_COM_3P3 (I/O), 3TPUFZP18_M1_COM_3P3 (I/O), 3TPUFZP18_M2_IND_3P3 (I/O), 3TPUFZP18_M1_IND_3P3 (I/O), HYPDFZP18_M2_IND_3P3 (I/O), HYPDFZP18_M1_IND_3P3 (I/O), HYPDFZP18_M2_COM_3P3 (I/O), HYPDFZP18_M1_COM_3P3 (I/O), BT3350BSHYPUFZP18_Z (I/O), BT3350BSHYPUFZP18_PU (I/O), BCHYPUFZP18M2IND3P3 (I/O), BCHYPUFZP18M1IND3P3 (I/O), BCHYPUFZP18M2COM3P3 (I/O), BCHYPUFZP18M1COM3P3 (I/O), PDFZSCP18_M1_IND_3P3 (I/O), PDFZSCP18_M5_IND_3P3 (I/O), PDFZSCP18_M1_COM_3P3 (I/O), PDFZSCP18_M5_COM_3P3 (I/O), PUFZSCP18_M1_IND_3P3 (I/O), PUFZSCP18_M5_IND_3P3 (I/O), PUFZSCP18_M1_COM_3P3 (I/O), PUFZSCP18_M5_COM_3P3 (I/O), FS (Output), LS (Output), HS (Output), FS_IN (Input), LS_IN (Input), KP18PUSR50_MODE2_M1 (Input), KP18PUSR50_MODE1_M1 (Input), KP18PUSR50_MODE2_M2 (Input), KP18PUSR50_MODE1_M2 (Input), SHYPDFZP18_MODE2_M1 (Input), SHYPDFZP18_MODE1_M1 (Input), SHYPDFZP18_MODE2_M2 (Input), SHYPDFZP18_MODE1_M2 (Input), SHYPUFZP18_MODE2_M1 (Input), SHYPUFZP18_MODE1_M1 (Input), SHYPUFZP18_MODE2_M2 (Input), SHYPUFZP18_MODE1_M2 (Input), BUF_MODE3_3P3_IND (3-state), BUF_MODE3_3P3_COM (3-state), OT3350BSFZP18_M1 (3-state), OT3350BSFZP18_M2 (3-state), OT3350CSFZP18_M1 (3-state), OT3350CSFZP18_M2 (3-state), BUF8_MODE1_3P3_IND (I/O), BUF8_MODE1_3P3_COM (I/O), NO_SR0_NO_TERM_1P8 (I/O), NO_TERM_1P8 (Input), SR0_NO_TERM_1P8 (I/O)
